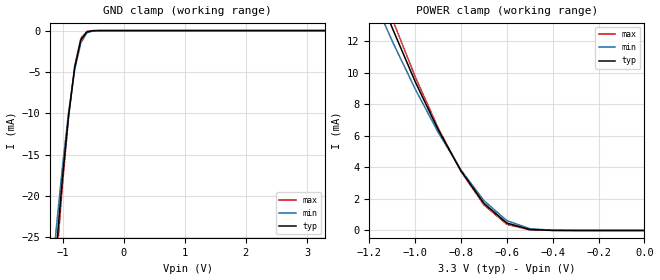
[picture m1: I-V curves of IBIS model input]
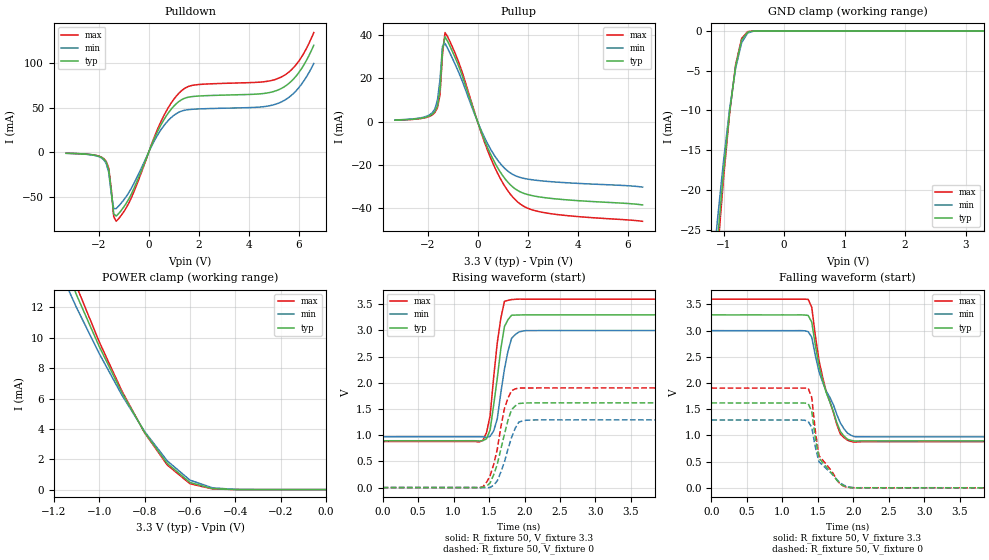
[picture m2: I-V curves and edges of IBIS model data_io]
[IBIS Ver]   3.2
[Comment Char]   |_char
[File name]   as7c34098a_tsopc.ibs
[File Rev]   1.1
[Date]   July 29, 2004 10:10:13 AM
[Source]
Alliance Semiconductor Corporation.
[Notes]
This model  is for TSOP package & Commercial operation.
[Disclaimer]
Data is for modelling purpose only & not guaranteed.
[Copyright]
Alliance Semiconductor Corporation
| TSOP Package
[Component]   7c34098a_tsopc
Si_location Pin
Timing_location Pin
[Manufacturer]   Alliance Semiconductor Corporation
[Package]
R_pkg   310m   170.7m   426.1m
L_pkg   4.9nH   3.2nH   6.505nH
C_pkg   0.9pF   0.51pF   1.215pF
[Pin] signal_name   model_name
1   A0   input
2   A1   input
3   A2   input
4   A3   input
5   A4   input
6   NCE   input
7   IO1   data_io
8   IO2   data_io
9   IO3   data_io
10   IO4   data_io
11   VCC   POWER
12   GND   GND
13   IO5   data_io
14   IO6   data_io
15   IO7   data_io
16   IO8   data_io
17   NWE   input
18   A5   input
19   A6   input
20   A7   input
21   A8   input
22   A9   input
23   A10   input
24   A11   input
25   A12   input
26   A13   input
27   A14   input
28   NC   NC
29   IO9   data_io
30   IO10   data_io
31   IO11   data_io
32   IO12   data_io
33   VCC   POWER
34   GND   GND
35   IO13   data_io
36   IO14   data_io
37   IO15   data_io
38   IO16   data_io
39   NLB   input
40   NUB   input
41   NOE   input
42   A15   input
43   A16   input
44   A17   input
| Models and submodels in the file (2): input (Input), data_io (I/O)
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[Model]   input
Model_type Input
Vinh=2V
Vinl=0.8V
C_comp   4.5pF   4.5pF   4.5pF
[Temperature Range] 25   70   0
[Voltage Range]   3.3   3.0   3.6
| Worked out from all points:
|   GND clamp passes 1 mA (typ) near -0.69 V on its own axis
|   POWER clamp passes 1 mA (typ) near -0.64 V on its own axis
[GND Clamp]
-3.3V     -5.963A    -5.809A    -6.051A
-1.2V     -35.86mA   -31.87mA   -38.5mA
-1.1V     -26.38mA   -23.79mA   -28.07mA
-1V       -17.75mA   -16.39mA   -18.6mA
-900mV    -10.25mA   -9.881mA   -10.45mA
-800mV    -4.452mA   -4.697mA   -4.259mA
-700mV    -1.141mA   -1.475mA   -944.5uA
-600mV    -151uA     -269.4uA   -100.2uA
-500mV    -13.23uA   -33.93uA   -6.772uA
-400mV    -845.7nA   -3.334uA   -320.1nA
3.3V      69.07pA    1.24uA     58.58pA
[POWER Clamp]
-3.3V     5.963A     5.808A     6.051A
-1.2V     16.57mA    15.3mA     17.44mA
-1.1V     12.83mA    11.99mA    13.4mA
-1V       9.429mA    8.967mA    9.743mA
-900mV    6.388mA    6.227mA    6.498mA
-800mV    3.775mA    3.828mA    3.742mA
-700mV    1.722mA    1.89mA     1.618mA
-600mV    472uA      624uA      388.6uA
-500mV    61.49uA    114.3uA    39.9uA
-400mV    5.003uA    13.47uA    2.506uA
0V        69.07pA    127.6pA    72.37pA
[Model]   data_io
Model_type I/O
Enable Active-High
Polarity Non-Inverting
Vinh=2V
Vinl=0.8V
Vref=1.728V
Vmeas=1.5V
Rref=168
Cref=5pF
C_comp   4.5pF   4.5pF   4.5pF
[Temperature Range] 25   70   0
[Voltage Range]   3.3   3.0   3.6
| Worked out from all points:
|   slope of the pulldown table from 0 to 0.495 V, typ, clamps not added: 16 ohm
|   slope of the pullup table from 0 to 0.495 V, typ, clamps not added: 34.3 ohm
|   GND clamp passes 1 mA (typ) near -0.69 V on its own axis
|   POWER clamp passes 1 mA (typ) near -0.64 V on its own axis
|   falling waveform, R_fixture 50, V_fixture 3.3: 20-80 % time 283ps typ, 319ps min, 271ps max; typ from 3.3 V to 0.895 V
|   falling waveform, R_fixture 50, V_fixture 0: 20-80 % time 236ps typ, 273ps min, 228ps max; typ from 1.62 V to 0.001 V
|   rising waveform, R_fixture 50, V_fixture 3.3: 20-80 % time 142ps typ, 143ps min, 128ps max; typ from 0.894 V to 3.3 V
|   rising waveform, R_fixture 50, V_fixture 0: 20-80 % time 184ps typ, 185ps min, 169ps max; typ from 0 V to 1.62 V
[Pullup]
-3.3V     659uA      743uA      615uA
-1.7V     4.782mA    5.917mA    4.251mA
-1.6V     7.4mA      10.09mA    6.437mA
-1.5V     14.72mA    19.44mA    12.4mA
-1.4V     33.46mA    34.75mA    31.23mA
-1.3V     39.19mA    36.13mA    41.17mA
-700mV    23.99mA    21.3mA     25.75mA
400mV     -11.98mA   -10.18mA   -13.27mA
900mV     -23.18mA   -19.28mA   -26.13mA
1.5V      -31.11mA   -25.01mA   -36.09mA
2.7V      -35.24mA   -27.6mA    -42.22mA
6.6V      -38.58mA   -30.34mA   -46.16mA
[Pulldown]
-3.3V     -1.242mA   -1.31mA    -1.211mA
-2.1V     -3.793mA   -4.121mA   -3.644mA
-1.7V     -11.14mA   -12.71mA   -10.39mA
-1.6V     -19.38mA   -22.76mA   -17.85mA
-1.4V     -69.26mA   -63.48mA   -72.43mA
-1.3V     -71.81mA   -63.34mA   -77.64mA
-700mV    -47.31mA   -40.82mA   -51.56mA
500mV     31.19mA    25.64mA    35.02mA
1.3V      58.66mA    45.99mA    68.69mA
5.3V      71.48mA    56.33mA    84.34mA
6V        89.27mA    72.35mA    102.2mA
6.6V      120mA      99.57mA    134.3mA
[GND Clamp]
-3.3V     -5.963A    -5.809A    -6.051A
-1.2V     -35.86mA   -31.87mA   -38.5mA
-1.1V     -26.38mA   -23.79mA   -28.07mA
-1V       -17.75mA   -16.39mA   -18.6mA
-900mV    -10.25mA   -9.881mA   -10.45mA
-800mV    -4.452mA   -4.697mA   -4.259mA
-700mV    -1.141mA   -1.475mA   -944.5uA
-600mV    -151uA     -269.4uA   -100.2uA
-500mV    -13.23uA   -33.93uA   -6.772uA
-400mV    -845.7nA   -3.334uA   -320.1nA
3.3V      69.07pA    1.24uA     58.58pA
[POWER Clamp]
-3.3V     5.963A     5.808A     6.051A
-1.2V     16.57mA    15.3mA     17.44mA
-1.1V     12.83mA    11.99mA    13.4mA
-1V       9.429mA    8.967mA    9.743mA
-900mV    6.388mA    6.227mA    6.498mA
-800mV    3.775mA    3.828mA    3.742mA
-700mV    1.722mA    1.89mA     1.618mA
-600mV    472uA      624uA      388.6uA
-500mV    61.49uA    114.3uA    39.9uA
-400mV    5.003uA    13.47uA    2.506uA
0V        69.07pA    127.6pA    72.37pA
[Falling Waveform]
R_fixture=50
V_fixture=3.3
V_fixture_min=3.0
V_fixture_max=3.6
0s        3.3V       3V         3.6V
1.364ns   3.289V     2.98V      3.596V
1.414ns   3.16V      2.872V     3.444V
1.515ns   2.334V     2.224V     2.438V
1.616ns   1.823V     1.848V     1.845V
1.717ns   1.46V      1.591V     1.446V
1.818ns   1.072V     1.235V     1.026V
1.919ns   925.9mV    1.042V     907.4mV
2.02ns    892.1mV    974.8mV    871.1mV
5ns       895.3mV    971.9mV    881.1mV
[Falling Waveform]
R_fixture=50
V_fixture=0
V_fixture_min=0
V_fixture_max=0
0s        1.619V     1.294V     1.904V
1.263ns   1.619V     1.294V     1.903V
1.364ns   1.606V     1.269V     1.902V
1.414ns   1.457V     1.15V      1.723V
1.465ns   949.4mV    778mV      1.085V
1.515ns   569.1mV    498mV      614.4mV
1.667ns   324.6mV    308.2mV    366.3mV
1.818ns   70.45mV    88.26mV    64.61mV
1.919ns   10.54mV    20.09mV    5.356mV
5ns       903uV      751.5uV    701uV
[Rising Waveform]
R_fixture=50
V_fixture=3.3
V_fixture_min=3.0
V_fixture_max=3.6
0s        894mV      970.6mV    879.7mV
1.414ns   897.3mV    969.2mV    905.5mV
1.465ns   931.9mV    956.5mV    1.05V
1.515ns   1.101V     979mV      1.374V
1.566ns   1.582V     1.084V     2.114V
1.616ns   2.091V     1.316V     2.768V
1.717ns   3.076V     2.263V     3.556V
1.818ns   3.293V     2.852V     3.591V
1.97ns    3.298V     2.988V     3.599V
5ns       3.299V     2.999V     3.599V
[Rising Waveform]
R_fixture=50
V_fixture=0
V_fixture_min=0
V_fixture_max=0
0s        0V         0V         0V
1.414ns   4.37mV     171.6uV    16.53mV
1.515ns   89.09mV    4.206mV    225.8mV
1.616ns   445.6mV    129.1mV    730.6mV
1.717ns   1.019V     492.6mV    1.512V
1.818ns   1.489V     960.2mV    1.852V
1.869ns   1.559V     1.134V     1.883V
1.919ns   1.605V     1.25V      1.903V
2.071ns   1.617V     1.289V     1.902V
5ns       1.619V     1.293V     1.903V
[Ramp]
R_load=50
dV/dt_r   9.712E-1/1.779E-10   7.760E-1/1.848E-10   1.142E+0/1.689E-10
dV/dt_f   1.443E+0/2.832E-10   1.217E+0/3.183E-10   1.631E+0/2.710E-10
|[End   data_io
